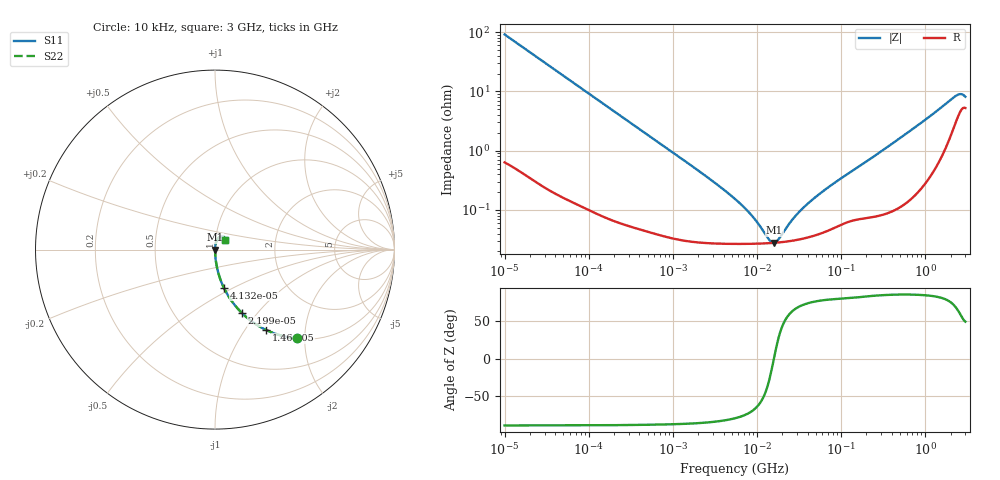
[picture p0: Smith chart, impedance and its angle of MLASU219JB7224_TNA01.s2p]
! MLASU219JB7224_TNA01  S-PARAMETER MODEL  ( Standard Model )
! Model Generated by TAIYO YUDEN Corporation (http://www.ty-top.com)
! Version 1.0
! TAIYO YUDEN Control No. 220601
! Copyright(c) 2011 TAIYO YUDEN CO.,LTD. All Rights Reserved.
! Product Description (link to TY-COMPAS)
! https://ds.yuden.co.jp/TYCOMPAS/or/detail?pn=MLASU219JB7224KTNA01&u=M
! Products Name : Multilayer Ceramic Capacitors
! Characteristics :
!  Capacitance : 0.22 [uF] , Rated Voltage : 50 [V] , TCC : X7R
!  Case Size : 2.0 x 1.25 / 0.079 x 0.049 [mm/inch] , Thickness : 0.85 / 0.033 [mm/inch]
!  (Conditions: Temperature = 25 [degC] , DC Bias Voltage = 0 [V])
! External Node Assignments :
!  1  o---| |---o  2
! GND o---------o GND
! Frequency Range : 10kHz  -  3GHz  [ 401 STEP ]
# MHZ S RI R 50
! Freq[MHz].  S11 Real  S11 Imag  S21 Real  S21 Imag  S12 Real  S12 Imag  S22 Real  S22 Imag
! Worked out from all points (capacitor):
!   401 points, 10 kHz to 3 GHz, reference 50 ohm
!   read as one part in series: C = 174 nF near 10.65 kHz
!   lowest |Z| = 27.9 mohm at 16 MHz (marker M1)
!   series resonance near 15.88 MHz, so ESL is about 580 pH
!   S11 on the Smith chart (normalised r, x): 10 kHz: 1.01, -1.83; 14.6 kHz: 1.01, -1.25; 22 kHz: 1.01, -0.83; 41.32 kHz: 1.00, -0.45; 3 GHz: 1.11, +0.12
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0.01  0.4556 -0.4946  0.5444 0.4946  0.5444 0.4946  0.4556 -0.4946
0.014599  0.284 -0.4472  0.716 0.4472  0.716 0.4472  0.284 -0.4472
0.021995  0.1502 -0.3535  0.8498 0.3535  0.8498 0.3535  0.1502 -0.3535
0.041322  0.0488 -0.2114  0.9512 0.2114  0.9512 0.2114  0.0488 -0.2114
0.082683  0.0134 -0.11  0.9866 0.11  0.9866 0.11  0.0134 -0.11
0.199902  0.00279 -0.0462  0.9972 0.0462  0.9972 0.0462  0.00279 -0.0462
0.683653  0.000565 -0.0136  0.9994 0.0136  0.9994 0.0136  0.000565 -0.0136
2.652321  0.000287 -0.00344  0.9997 0.00344  0.9997 0.00344  0.000287 -0.00344
5.477226  0.00027 -0.00151  0.9997 0.00151  0.9997 0.00151  0.00027 -0.00151
8.789267  0.000269 -0.000741  0.9997 0.000741  0.9997 0.000741  0.000269 -0.000741
14.10408  0.000276 -0.00014  0.9997 0.00014  0.9997 0.00014  0.000276 -0.00014
15.99985  0.000279 9.14e-06  0.9997 -9.14e-06  0.9997 -9.14e-06  0.000279 9.14e-06
18.15044  0.000283 0.000158  0.9997 -0.000158  0.9997 -0.000158  0.000283 0.000158
24.10585  0.000297 0.000503  0.9997 -0.000503  0.9997 -0.000503  0.000297 0.000503
29.12589  0.000311 0.000752  0.9997 -0.000752  0.9997 -0.000752  0.000311 0.000752
45.28751  0.000362 0.00144  0.9996 -0.00144  0.9996 -0.00144  0.000362 0.00144
82.4407  0.000503 0.00279  0.9995 -0.00279  0.9995 -0.00279  0.000503 0.00279
374.4521  0.00105 0.0121  0.9989 -0.0121  0.9989 -0.0121  0.00105 0.0121
1321.625  0.00699 0.0441  0.993 -0.0441  0.993 -0.0441  0.00699 0.0441
2188.735  0.0294 0.072  0.9706 -0.072  0.9706 -0.072  0.0294 0.072
2562.461  0.047 0.072  0.953 -0.072  0.953 -0.072  0.047 0.072
3000  0.0532 0.0558  0.9468 -0.0558  0.9468 -0.0558  0.0532 0.0558
